| IBIS file created by T2B Version 16.0.0.01291   000
| Cadence Design Systems, Inc. 2011
| Simulator:  ****** HSPICE -- O-2018.09-1 win64 (Sep 27 2018) ******
| This Model is valid for Automotive grade 1 Temperature Range -40C<=Tc<=125C
| Valid for LPDDR2-1066 operation
| Part Number   VDD2/VDDQ   Package   Architecture
| SCB4BL1G320AF-19GA1   1.2 +0.1/-0.06  BGA178   32Meg x 32
| SCB4BL1G160AF-19GA1   1.2 +0.1/-0.06  BGA178   64Meg x 16
[IBIS ver] 5.0
[File name]  usssl1gxxaa1.ibs
[File Rev]  1.0
[Date]   September 8, 2021
[Source] Simulation of a silicon level SPICE model
[Notes]  IBIS Characteristics for I/O Buffer
  IBIS Model Revision History:
  Rev 1.0:  2021-09-08 - IBIS model file initial creation
[Disclaimer]  The IBIS models are for modeling purpose only and are subject to change without any notice. UniIC is not
  responsible for any problems the models may cause.
[Copyright] Copyright 2021 UniIC Semiconductors Corp. All rights reserved
|   Component SCB4BL1G320AF-19GA1
[Component] SCB4BL1G320AF-19GA1
[Manufacturer] UniIC Semiconductors Corp.
[Package]
| variable   typ   min   max
R_pkg   0.856   0.666   0.979
L_pkg   3.510nH   2.420nH   3.790nH
C_pkg   0.923pF   0.659pF   1.120pF
[Pin]  signal_name   model_name   R_pin   L_pin   C_pin
A1   NC1   NC   NA   NA   NA
A2   NC2   NC   NA   NA   NA
A3   VDD1   Power   NA   NA   NA
A4   VDD1   Power   NA   NA   NA
A5   VDD1   Power   NA   NA   NA
A6   VDD1   Power   NA   NA   NA
A8   VDD2   Power   NA   NA   NA
A9   VDD2   Power   NA   NA   NA
A10   VDD1   Power   NA   NA   NA
A11   VDDQ   Power   NA   NA   NA
A12   NC3   NC   NA   NA   NA
A13   NC4   NC   NA   NA   NA
B1   NC5   NC   NA   NA   NA
B2   VSS   Gnd   NA   NA   NA
B3   ZQ   Power   NA   NA   NA
B4   ZQ1   Power   NA   NA   NA
B5   VSS   Gnd   NA   NA   NA
B6   VSS   Gnd   NA   NA   NA
B8   DQ31   DQ   0.960   3.760nH   0.966pF
B9   DQ30   DQ   0.854   3.760nH   0.813pF
B10   DQ29   DQ   0.856   3.610nH   0.783pF
B11   DQ28   DQ   0.960   3.760nH   0.966pF
B12   VSS   Gnd   NA   NA   NA
B13   NC7   NC   NA   NA   NA
C2   CA9   CA   0.698   2.600nH   0.708pF
C3   VSS   Gnd   NA   NA   NA
C4   NC8   NC   NA   NA   NA
C5   VSS   Gnd   NA   NA   NA
C6   VSS   Gnd   NA   NA   NA
C8   DQ27   DQ   0.917   3.660nH   0.933pF
C9   DQ26   DQ   0.792   3.450nH   0.792pF
C10   DQ25   DQ   0.782   3.450nH   0.759pF
C11   DQ23   DQ   0.862   3.460nH   0.862pF
C12   VDDQ   Power   NA   NA   NA
D2   CA8   CA   0.659   2.440nH   0.679pF
D3   VSS   Gnd   NA   NA   NA
D4   VDD2   Power   NA   NA   NA
D5   VDD2   Power   NA   NA   NA
D6   VDD2   Power   NA   NA   NA
D8   DM3   DQ   0.872   3.490nH   0.997pF
D9   DQ15   DQ   0.881   3.570nH   0.999pF
D10   DQS3_T   DQ   0.784   3.080nH   0.869pF
D11   DQS3_C   DQ   0.754   3.120nH   0.829pF
D12   VSS   Gnd   NA   NA   NA
E2   CA7   CA   0.654   2.420nH   0.681pF
E3   CA6   CA   0.717   2.660nH   0.758pF
E4   VSS   Gnd   NA   NA   NA
E5   VSS   Gnd   NA   NA   NA
E6   VSS   Gnd   NA   NA   NA
E8   VDDQ   Power   NA   NA   NA
E9   DQ14   DQ   0.832   3.400nH   0.898pF
E10   DQ13   DQ   0.812   3.330nH   0.925pF
E11   DQ12   DQ   0.837   3.220nH   0.921pF
E12   VDDQ   Power   NA   NA   NA
F2   VDD2   Power   NA   NA   NA
F3   CA5   CA   0.667   2.530nH   0.681pF
F4   VSS   Gnd   NA   NA   NA
F5   VSS   Gnd   NA   NA   NA
F6   VSS   Gnd   NA   NA   NA
F8   DQ11   DQ   0.863   3.250nH   0.978pF
F9   DQ10   DQ   0.801   3.100nH   0.918pF
F10   DQ9   DQ   0.830   3.120nH   0.968pF
F11   DQ8   DQ   0.858   3.270nH   0.978pF
F12   VSS   Gnd   NA   NA   NA
G2   VDD2   Power   NA   NA   NA
G3   VSS   Gnd   NA   NA   NA
G4   VSS   Gnd   NA   NA   NA
G5   VDD2   Power   NA   NA   NA
G6   VSS   Gnd   NA   NA   NA
G8   DM1   DQ   0.820   3.100nH   0.987pF
G9   VSS   Gnd   NA   NA   NA
G10   DQS1_T   DQ   0.798   2.950nH   0.934pF
G11   DQS1_C   DQ   0.793   2.940nH   0.945pF
G12   VDD2   Power   NA   NA   NA
H2   VSS   Gnd   NA   NA   NA
H3   VDD2   Power   NA   NA   NA
H4   VREFCA   Power   NA   NA   NA
H5   VDD2   Power   NA   NA   NA
H6   VDD2   Power   NA   NA   NA
H7   VDDQ   Power   NA   NA   NA
H8   VDDQ   Power   NA   NA   NA
H9   VDDQ   Power   NA   NA   NA
H10   VSS   Gnd   NA   NA   NA
H11   VDDQ   Power   NA   NA   NA
H12   VDD2   Power   NA   NA   NA
J2   CK_C   CA   0.699   2.690nH   0.684pF
J3   CK_T   CA   0.694   2.490nH   0.738pF
J4   VSS   Gnd   NA   NA   NA
J5   VDD2   Power   NA   NA   NA
J6   VDD2   Power   NA   NA   NA
J8   ODT   DQ   0.960   3.760nH   0.966pF
J9   VDDQ   Power   NA   NA   NA
J10   VDDQ   Power   NA   NA   NA
J11   VREFDQ   Power   NA   NA   NA
J12   VSS   Gnd   NA   NA   NA
K2   VSS   Gnd   NA   NA   NA
K3   CKE   CKE   0.765   2.850nH   0.710pF
K4   CKE1   CKE   0.765   2.850nH   0.710pF
K5   VDD2   Power   NA   NA   NA
K6   VDD2   Power   NA   NA   NA
K8   VDDQ   Power   NA   NA   NA
K9   NC10   NC   NA   NA   NA
K10   VSS   Gnd   NA   NA   NA
K11   VDDQ   Power   NA   NA   NA
K12   VDD2   Power   NA   NA   NA
L2   VDD2   Power   NA   NA   NA
L3   CS_N   CA   0.666   2.580nH   0.659pF
L4   CS1_N   CA   0.666   2.580nH   0.659pF
L5   VDD2   Power   NA   NA   NA
L6   VSS   Gnd   NA   NA   NA
L8   DM0   DQ   0.867   2.930nH   1.012pF
L9   VSS   Gnd   NA   NA   NA
L10   DQS0_T   DQ   0.735   2.640nH   0.875pF
L11   DQS0_C   DQ   0.743   2.680nH   0.926pF
L12   VDDQ   Power   NA   NA   NA
M2   VDD2   Power   NA   NA   NA
M3   CA4   CA   0.693   2.670nH   0.671pF
M4   VSS   Gnd   NA   NA   NA
M5   VSS   Gnd   NA   NA   NA
M6   VSS   Gnd   NA   NA   NA
M8   DQ4   DQ   0.888   3.410nH   0.989pF
M9   DQ5   DQ   0.801   3.240nH   0.903pF
M10   DQ6   DQ   0.774   3.190nH   0.897pF
M11   DQ7   DQ   0.813   3.110nH   0.911pF
M12   VSS   Gnd   NA   NA   NA
N2   CA2   CA   0.685   2.540nH   0.695pF
N3   CA3   CA   0.732   2.700nH   0.728pF
N4   VSS   Gnd   NA   NA   NA
N5   VSS   Gnd   NA   NA   NA
N6   VSS   Gnd   NA   NA   NA
N8   VDDQ   Power   NA   NA   NA
N9   DQ1   DQ   0.817   3.620nH   0.822pF
N10   DQ2   DQ   0.797   3.290nH   0.873pF
N11   DQ3   DQ   0.778   3.120nH   0.866pF
N12   VDDQ   Power   NA   NA   NA
P2   CA1   CA   0.765   2.810nH   0.746pF
P3   VSS   Gnd   NA   NA   NA
P4   VDD2   Power   NA   NA   NA
P5   VDD2   Power   NA   NA   NA
P6   VDD2   Power   NA   NA   NA
P8   DM2   DQ   0.860   3.610nH   0.972pF
P9   DQ1   DQ   0.817   3.620nH   0.822pF
P10   DQS2_T   DQ   0.835   3.400nH   0.827pF
P11   DQS2_C   DQ   0.775   3.350nH   0.836pF
P12   VSS   Gnd   NA   NA   NA
R2   CA0   CA   0.832   3.090nH   0.766pF
R3   TBI   Power   NA   NA   NA
R4   VSS   Gnd   NA   NA   NA
R5   VSS   Gnd   NA   NA   NA
R6   VSS   Gnd   NA   NA   NA
R8   DQ20   DQ   0.916   3.920nH   0.957pF
R9   DQ21   DQ   0.854   3.760nH   0.847pF
R10   DQ22   DQ   0.828   3.640nH   0.832pF
R11   DQ23   DQ   0.862   3.460nH   0.816pF
R12   VDDQ   Power   NA   NA   NA
T1   NC12   NC   NA   NA   NA
T2   VSS   Gnd   NA   NA   NA
T3   VSS   Gnd   NA   NA   NA
T4   VSS   Gnd   NA   NA   NA
T5   VSS   Gnd   NA   NA   NA
T6   VSS   Gnd   NA   NA   NA
T8   DQ16   DQ   0.979   3.870nH   0.990pF
T9   DQ17   DQ   0.891   3.870nH   0.893pF
T10   DQ18   DQ   0.856   3.790nH   0.838pF
T11   DQ19   DQ   0.892   3.720nH   0.852pF
T12   VDD1   Power   NA   NA   NA
T13   NC13   NC   NA   NA   NA
U1   NC14   NC   NA   NA   NA
U2   NC15   NC   NA   NA   NA
U3   VDD1   Power   NA   NA   NA
U4   VDD1   Power   NA   NA   NA
U5   VDD1   Power   NA   NA   NA
U6   VDD1   Power   NA   NA   NA
U8   VDD2   Power   NA   NA   NA
U9   VDD2   Power   NA   NA   NA
U10   VDD1   Power   NA   NA   NA
U11   VDDQ   Power   NA   NA   NA
U12   NC16   NC   NA   NA   NA
U13   NC17   NC   NA   NA   NA
|IN   dq_in   dummy
|EN   dq_en   dummy
[Diff pin]  inv_pin  vdiff   tdelay_typ   tdelay_min   tdelay_max
D10   D11   0.300V   NA   NA   NA
G10   G11   0.300V   NA   NA   NA
J2   J3   0.300V   NA   NA   NA
L10   L11   0.300V   NA   NA   NA
P10   P11   0.300V   NA   NA   NA
|   Component SCB4BL1G160AF-19GA1
[Component] SCB4BL1G160AF-19GA1
[Manufacturer] UniIC Semiconductors Corp.
[Package]
| variable   typ   min   max
R_pkg   0.856   0.666   0.979
L_pkg   3.510nH   2.420nH   3.790nH
C_pkg   0.923pF   0.659pF   1.120pF
[Pin]  signal_name   model_name   R_pin   L_pin   C_pin
A1   NC1   NC   NA   NA   NA
A2   NC2   NC   NA   NA   NA
A3   VDD1   Power   NA   NA   NA
A4   VDD1   Power   NA   NA   NA
A5   VDD1   Power   NA   NA   NA
A6   VDD1   Power   NA   NA   NA
A8   VDD2   Power   NA   NA   NA
A9   VDD2   Power   NA   NA   NA
A10   VDD1   Power   NA   NA   NA
A11   VDDQ   Power   NA   NA   NA
A12   NC3   NC   NA   NA   NA
A13   NC4   NC   NA   NA   NA
B1   NC5   NC   NA   NA   NA
B2   VSS   Gnd   NA   NA   NA
B3   ZQ   Power   NA   NA   NA
B4   ZQ1   Power   NA   NA   NA
B5   VSS   Gnd   NA   NA   NA
B6   VSS   Gnd   NA   NA   NA
B8   NC18   NC   NA   NA   NA
B9   NC19   NC   NA   NA   NA
B10   NC20   NC   NA   NA   NA
B11   NC21   NC   NA   NA   NA
B12   VSS   Gnd   NA   NA   NA
B13   NC7   NC   NA   NA   NA
C2   CA9   CA   0.698   2.600nH   0.708pF
C3   VSS   Gnd   NA   NA   NA
C4   NC8   NC   NA   NA   NA
C5   VSS   Gnd   NA   NA   NA
C6   VSS   Gnd   NA   NA   NA
C8   NC22   NC   NA   NA   NA
C9   NC23   NC   NA   NA   NA
C10   NC24   NC   NA   NA   NA
C11   NC25   NC   NA   NA   NA
C12   VDDQ   Power   NA   NA   NA
D2   CA8   CA   0.659   2.440nH   0.679pF
D3   VSS   Gnd   NA   NA   NA
D4   VDD2   Power   NA   NA   NA
D5   VDD2   Power   NA   NA   NA
D6   VDD2   Power   NA   NA   NA
D8   NC26   NC   NA   NA   NA
D9   DQ15   DQ   0.881   3.570nH   0.999pF
D10   NC27   NC   NA   NA   NA
D11   NC28   NC   NA   NA   NA
D12   VSS   Gnd   NA   NA   NA
E2   CA7   CA   0.654   2.420nH   0.681pF
E3   CA6   CA   0.717   2.660nH   0.758pF
E4   VSS   Gnd   NA   NA   NA
E5   VSS   Gnd   NA   NA   NA
E6   VSS   Gnd   NA   NA   NA
E8   VDDQ   Power   NA   NA   NA
E9   DQ14   DQ   0.832   3.400nH   0.898pF
E10   DQ13   DQ   0.812   3.330nH   0.925pF
E11   DQ12   DQ   0.837   3.220nH   0.921pF
E12   VDDQ   Power   NA   NA   NA
F2   VDD2   Power   NA   NA   NA
F3   CA5   CA   0.667   2.530nH   0.681pF
F4   VSS   Gnd   NA   NA   NA
F5   VSS   Gnd   NA   NA   NA
F6   VSS   Gnd   NA   NA   NA
F8   DQ11   DQ   0.863   3.250nH   0.978pF
F9   DQ10   DQ   0.801   3.100nH   0.918pF
F10   DQ9   DQ   0.830   3.120nH   0.968pF
F11   DQ8   DQ   0.858   3.270nH   0.978pF
F12   VSS   Gnd   NA   NA   NA
G2   VDD2   Power   NA   NA   NA
G3   VSS   Gnd   NA   NA   NA
G4   VSS   Gnd   NA   NA   NA
G5   VDD2   Power   NA   NA   NA
G6   VSS   Gnd   NA   NA   NA
G8   DM1   DQ   0.820   3.100nH   0.987pF
G9   VSS   Gnd   NA   NA   NA
G10   DQS1_T   DQ   0.798   2.950nH   0.934pF
G11   DQS1_C   DQ   0.793   2.940nH   0.945pF
G12   VDD2   Power   NA   NA   NA
H2   VSS   Gnd   NA   NA   NA
H3   VDD2   Power   NA   NA   NA
H4   VREFCA   Power   NA   NA   NA
H5   VDD2   Power   NA   NA   NA
H6   VDD2   Power   NA   NA   NA
H7   VDDQ   Power   NA   NA   NA
H8   VDDQ   Power   NA   NA   NA
H9   VDDQ   Power   NA   NA   NA
H10   VSS   Gnd   NA   NA   NA
H11   VDDQ   Power   NA   NA   NA
H12   VDD2   Power   NA   NA   NA
J2   CK_C   CA   0.699   2.690nH   0.684pF
J3   CK_T   CA   0.694   2.490nH   0.738pF
J4   VSS   Gnd   NA   NA   NA
J5   VDD2   Power   NA   NA   NA
J6   VDD2   Power   NA   NA   NA
J8   ODT   DQ   0.960   3.760nH   0.966pF
J9   VDDQ   Power   NA   NA   NA
J10   VDDQ   Power   NA   NA   NA
J11   VREFDQ   Power   NA   NA   NA
J12   VSS   Gnd   NA   NA   NA
K2   VSS   Gnd   NA   NA   NA
K3   CKE   CKE   0.765   2.850nH   0.710pF
K4   CKE1   CKE   0.765   2.850nH   0.710pF
K5   VDD2   Power   NA   NA   NA
K6   VDD2   Power   NA   NA   NA
K8   VDDQ   Power   NA   NA   NA
K9   NC10   NC   NA   NA   NA
K10   VSS   Gnd   NA   NA   NA
K11   VDDQ   Power   NA   NA   NA
K12   VDD2   Power   NA   NA   NA
L2   VDD2   Power   NA   NA   NA
L3   CS_N   CA   0.666   2.580nH   0.659pF
L4   CS1_N   CA   0.666   2.580nH   0.659pF
L5   VDD2   Power   NA   NA   NA
L6   VSS   Gnd   NA   NA   NA
L8   DM0   DQ   0.867   2.930nH   1.012pF
L9   VSS   Gnd   NA   NA   NA
L10   DQS0_T   DQ   0.735   2.640nH   0.875pF
L11   DQS0_C   DQ   0.743   2.680nH   0.926pF
L12   VDDQ   Power   NA   NA   NA
M2   VDD2   Power   NA   NA   NA
M3   CA4   CA   0.693   2.670nH   0.671pF
M4   VSS   Gnd   NA   NA   NA
M5   VSS   Gnd   NA   NA   NA
M6   VSS   Gnd   NA   NA   NA
M8   DQ4   DQ   0.888   3.410nH   0.989pF
M9   DQ5   DQ   0.801   3.240nH   0.903pF
M10   DQ6   DQ   0.774   3.190nH   0.897pF
M11   DQ7   DQ   0.813   3.110nH   0.911pF
M12   VSS   Gnd   NA   NA   NA
N2   CA2   CA   0.685   2.540nH   0.695pF
N3   CA3   CA   0.732   2.700nH   0.728pF
N4   VSS   Gnd   NA   NA   NA
N5   VSS   Gnd   NA   NA   NA
N6   VSS   Gnd   NA   NA   NA
N8   VDDQ   Power   NA   NA   NA
N9   DQ1   DQ   0.817   3.620nH   0.822pF
N10   DQ2   DQ   0.797   3.290nH   0.873pF
N11   DQ3   DQ   0.778   3.120nH   0.866pF
N12   VDDQ   Power   NA   NA   NA
P2   CA1   CA   0.765   2.810nH   0.746pF
P3   VSS   Gnd   NA   NA   NA
P4   VDD2   Power   NA   NA   NA
P5   VDD2   Power   NA   NA   NA
P6   VDD2   Power   NA   NA   NA
P8   NC29   NC   NA   NA   NA
P9   DQ1   DQ   0.817   3.620nH   0.822pF
P10   NC30   NC   NA   NA   NA
P11   NC31   NC   NA   NA   NA
P12   VSS   Gnd   NA   NA   NA
R2   CA0   CA   0.832   3.090nH   0.766pF
R3   TBI   Power   NA   NA   NA
R4   VSS   Gnd   NA   NA   NA
R5   VSS   Gnd   NA   NA   NA
R6   VSS   Gnd   NA   NA   NA
R8   NC32   NC   NA   NA   NA
R9   NC33   NC   NA   NA   NA
R10   NC34   NC   NA   NA   NA
R11   NC35   NC   NA   NA   NA
R12   VDDQ   Power   NA   NA   NA
T1   NC12   NC   NA   NA   NA
T2   VSS   Gnd   NA   NA   NA
T3   VSS   Gnd   NA   NA   NA
T4   VSS   Gnd   NA   NA   NA
T5   VSS   Gnd   NA   NA   NA
T6   VSS   Gnd   NA   NA   NA
T8   NC36   NC   NA   NA   NA
T9   NC37   NC   NA   NA   NA
T10   NC38   NC   NA   NA   NA
T11   NC39   NC   NA   NA   NA
T12   VDD1   Power   NA   NA   NA
T13   NC13   NC   NA   NA   NA
U1   NC14   NC   NA   NA   NA
U2   NC15   NC   NA   NA   NA
U3   VDD1   Power   NA   NA   NA
U4   VDD1   Power   NA   NA   NA
U5   VDD1   Power   NA   NA   NA
U6   VDD1   Power   NA   NA   NA
U8   VDD2   Power   NA   NA   NA
U9   VDD2   Power   NA   NA   NA
U10   VDD1   Power   NA   NA   NA
U11   VDDQ   Power   NA   NA   NA
U12   NC16   NC   NA   NA   NA
U13   NC17   NC   NA   NA   NA
[Diff pin]  inv_pin  vdiff   tdelay_typ   tdelay_min   tdelay_max
D10   D11   0.300V   NA   NA   NA
J2   J3   0.300V   NA   NA   NA
L10   L11   0.300V   NA   NA   NA
[Model Selector] DQ
DQ_RON240  RON=240ohms
DQ_RON120  RON=120ohms
DQ_RON80  RON=80ohms
DQ_RON60  RON=60ohms
DQ_RON48  RON=48ohms
DQ_RON40  RON=40ohms
DQ_RON34  RON=34ohms
DQ_RCV_ODTOFF  DQ_RCV_ODTOFF
DQ_RCV_ODT240  DQ_RCV_ODT240
DQ_RCV_ODT120  DQ_RCV_ODT120
DQ_RCV_ODT60  DQ_RCV_ODT60
| Models and submodels in the file (16): DQ_RON240 (I/O), DQ_RON120 (I/O), DQ_RON80 (I/O), DQ_RON60 (I/O), DQ_RON48 (I/O), DQ_RON40 (I/O), DQ_RON34 (I/O), DQ_RCV_ODTOFF (Input), DQ_RCV_ODT240 (Input), DQ_RCV_ODT120 (Input), DQ_RCV_ODT60 (Input), CA (Input), CKE (Input), DQ_ODT240 (Dynamic_clamp), DQ_ODT120 (Dynamic_clamp), DQ_ODT60 (Dynamic_clamp)
